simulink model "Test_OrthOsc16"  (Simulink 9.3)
settings: Solver=VariableStepAuto  StartTime=0.0  StopTime=0.4  RelTol=1e-3
InitFcn:
  | Test_LibVishia_Ctrl.TestOrthOsc_init()
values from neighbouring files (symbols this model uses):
  Orth_fb = 0    [stimuli_OrthBandpass.m]
  Orth_fqA = 50    [stimuli_OrthBandpass.m]
  Orth_fqB = 0    [stimuli_OrthBandpass.m]
  Orth_k0AB = 1    [stimuli_OrthBandpass.m]
  Orth_kA = 0.1    [stimuli_OrthBandpass.m]
  Orth_kB = 0    [stimuli_OrthBandpass.m]
  Tfq = 0.020    (= 0.02)    [TestOrthOsc_init.m]
  Tstep = 0.000050    (= 5e-05)    [TestOrthOsc_init.m]    (also in Test_PIDctrl_init.m = 0.0001)
libraries: libVishia_CtrlSfn x23, libVishia_Conv x16, libVishia_Ctrl x10, libVishia_Inspc x5, simulink x2

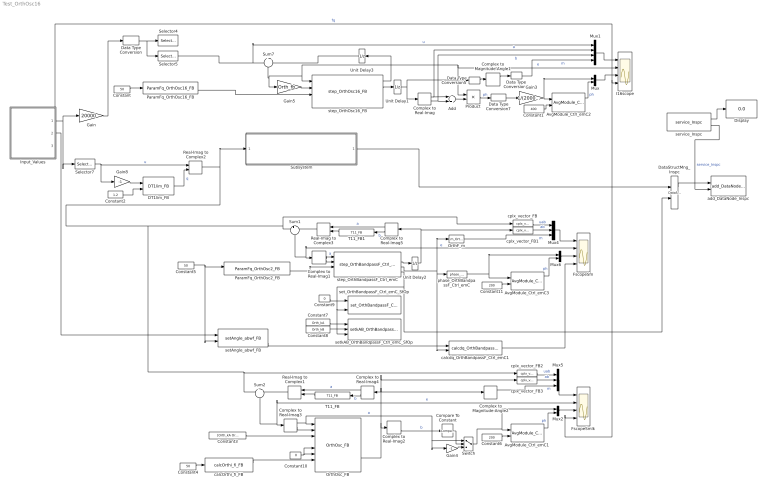
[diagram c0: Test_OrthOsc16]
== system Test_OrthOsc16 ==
  Add : Sum
  AvgModule_Ctrl_emC1 : libVishia_CtrlSfn/AvgModule_Ctrl_emC  SystemSampleTime=-1
  AvgModule_Ctrl_emC2 : libVishia_CtrlSfn/AvgModule_Ctrl_emC  SystemSampleTime=-1
  AvgModule_Ctrl_emC3 : libVishia_CtrlSfn/AvgModule_Ctrl_emC  SystemSampleTime=-1
  Compare To Constant : simulink/Logic and Bit Operations/Compare To Constant  relop=>=  const=0  OutDataTypeStr=boolean
  Complex to Magnitude-Angle1 : ComplexToMagnitudeAngle
  Complex to Magnitude-Angle2 : ComplexToMagnitudeAngle
  Complex to Real-Imag{,1..5} (6 alike) : ComplexToRealImag
  Constant : Constant  Value=50  OutDataTypeStr=single
  Constant1 : Constant  Value=400  OutDataTypeStr=single
  Constant10 : Constant  Value=0  OutDataTypeStr=boolean
  Constant11 : Constant  Value=200  OutDataTypeStr=single
  Constant2 : Constant  Value=1.2  OutDataTypeStr=single
  Constant3 : Constant  Value=[Orth_kA Orth_kB]  OutDataTypeStr=single
  Constant4 : Constant  Value=50  OutDataTypeStr=single
  Constant5 : Constant  Value=50  OutDataTypeStr=single
  Constant6 : Constant  Value=200  OutDataTypeStr=single
  Constant7 : Constant  Value=Orth_kA  OutDataTypeStr=single
  Constant8 : Constant  Value=Orth_kB  OutDataTypeStr=single
  Constant9 : Constant  Value=0  OutDataTypeStr=boolean
  DT1lim_FB : libVishia_Ctrl/DT1lim_FB  T1=0.0002  Td=0.02 / (2*pi)  Tstep=Tstep
  Data Type Conversion : DataTypeConversion  OutDataTypeStr=int16
  Data Type Conversion5 : DataTypeConversion  OutDataTypeStr=single
  Data Type Conversion6 : DataTypeConversion  OutDataTypeStr=int16
  Data Type Conversion7 : DataTypeConversion  OutDataTypeStr=single
  DataStructMng_Inspc : libVishia_Inspc/DataStructMng_Inspc  dirGenSource=''  typeData='Test_OrthBandpass'  inherit=off  chain=off  inputs=|
      | =f32: F32_Test_OrthBandpass;
      | =f: OrthBandpassF_Ctrl_emC;
  Display : Display
  FscopeSfn : Scope  NumInputPorts=4
  FscopeSmlk : Scope  NumInputPorts=4
  Gain : Gain  Gain=20000
  Gain3 : Gain  Gain=1/(20000*20000)
  Gain4 : Gain  Gain=-1
  Gain5 : Gain  Gain=Orth_fb
  Gain8 : Gain  Gain=-1
  I16scope : Scope  NumInputPorts=4
  Input_Values : Subsystem
  Mux : Mux  Inputs=2
  Mux1 : Mux
  Mux2 : Mux  Inputs=2
  Mux4 : Mux  Inputs=3
  Mux5 : Mux  Inputs=3
  Mux6 : Mux  Inputs=2
  OrthF_m : libVishia_CtrlSfn/m_OrthBandpass_Ctrl_emC  SystemSampleTime=-1
  OrthOsc_FB : libVishia_Ctrl/OrthOsc_FB
  ParamFq_OrthOsc16_FB : libVishia_CtrlSfn/ParamFq_OrthOsc16_FB  identObj=123  Tstep=16*Tstep  TstepOrth=Tstep  m_nom=100
  ParamFq_OrthOsc2_FB : libVishia_CtrlSfn/ParamFq_OrthOsc2_FB  identObj=123  Tstep=16*Tstep  TstepOrth=Tstep  m_nom=1.0
  Product : Product
  Real-Imag to Complex1 : RealImagToComplex
  Real-Imag to Complex2 : RealImagToComplex
  Real-Imag to Complex3 : RealImagToComplex
  Selector4 : Selector  IndexMode=Zero-based  InputPortWidth=2  IndexOptions=Index vector (dialog)  Indices=[0]  OutputSizes=1
  Selector5 : Selector  IndexMode=Zero-based  InputPortWidth=2  IndexOptions=Index vector (dialog)  Indices=[1]  OutputSizes=1
  Selector7 : Selector  IndexMode=Zero-based  InputPortWidth=2  IndexOptions=Index vector (dialog)  Indices=[1]  OutputSizes=1
  Subsystem : Subsystem
  Sum1 : Sum  Inputs=+|-
  Sum2 : Sum  Inputs=+|-
  Sum7 : Sum  Inputs=+|-
  Switch : Switch  Criteria=u2 > Threshold
  T11_FB : libVishia_Ctrl/T11_FB  T1=0.0002  y0=0  Tstep=Tstep
  T11_FB1 : libVishia_Ctrl/T11_FB  T1=0.0002  y0=0  Tstep=Tstep
  Unit Delay1 : UnitDelay  SampleTime=-1  HasFrameUpgradeWarning=on
  Unit Delay2 : UnitDelay  SampleTime=-1  HasFrameUpgradeWarning=on
  Unit Delay3 : UnitDelay  SampleTime=-1  HasFrameUpgradeWarning=on
  add_DataNode_Inspc : libVishia_Inspc/add_DataNode_Inspc  name1Refl='main'  name2Refl='_data'
  calcOrthi_fi_FB : libVishia_Ctrl/calcOrthi_fi_FB  Tstep=Tstep
  calcdq_OrthBandpassF_Ctrl_emC1 : libVishia_CtrlSfn/calcdq_OrthBandpassF_Ctrl_emC1  SystemSampleTime=-1
  cplx_vector_FB{,1..3} (4 alike) : libVishia_Conv/cplx_vector_FB  SystemSampleTime=-1
  phase_OrthBandpassF_Ctrl_emC : libVishia_CtrlSfn/phase_OrthBandpassF_Ctrl_emC  SystemSampleTime=-1
  service_Inspc : libVishia_Inspc/service_Inspc  Tstep=Tstep  IpPort='UDP:0.0.0.0:60094'
  setAngle_abwf_FB : libVishia_CtrlSfn/setAngle_abwf_FB  identObj=123  Tstep=Tstep
  set_OrthBandpassF_Ctrl_emC_SfOp : libVishia_CtrlSfn/set_OrthBandpassF_Ctrl_emC_SfOp  SystemSampleTime=-1
  setkAB_OrthBandpassF_Ctrl_emC_SfOp : libVishia_CtrlSfn/setkAB_OrthBandpassF_Ctrl_emC_SfOp  SystemSampleTime=-1
  step_OrthBandpassF_Ctrl_emC : libVishia_CtrlSfn/step_OrthBandpassF_Ctrl_emC  kA=1.0  kB=0
  step_OrthOsc16_FB : libVishia_CtrlSfn/step_OrthOsc16_FB  kA=Orth_kA  kB=Orth_kB
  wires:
  ParamFq_OrthOsc16_FB/2 -> step_OrthOsc16_FB/3
  Input_Values/1(Out1) -> Selector7/1, Gain/1
  Data Type Conversion/1 -> Selector5/1, Selector4/1
  Selector5/1 -> Sum7/1, Mux1/1  "u"
  Constant/1 -> ParamFq_OrthOsc16_FB/1
  Input_Values/2(Out2) -> setAngle_abwf_FB/1
  step_OrthOsc16_FB/2 -> Unit Delay1/1
  Add/1 -> Product/2
  Sum7/1 -> Gain5/1, step_OrthOsc16_FB/1, I16scope/2, Product/1  "e"
  Gain/1 -> Data Type Conversion/1
  Input_Values/3(Out3) -> FscopeSmlk/4, I16scope/4  "fq"
  Constant3/1 -> OrthOsc_FB/3
  calcOrthi_fi_FB/1 -> OrthOsc_FB/7
  Constant4/1 -> calcOrthi_fi_FB/1
  OrthOsc_FB/3 -> Complex to Magnitude-Angle2/1, cplx_vector_FB3/1, Complex to Real-Imag4/1, Complex to Real-Imag2/1
  Mux5/1 -> FscopeSmlk/1
  Complex to Real-Imag2/2 -> Compare To Constant/1  "b"
  Selector7/1 -> Real-Imag to Complex2/1, Gain8/1  "u"
  Switch/1 -> Mux2/1, AvgModule_Ctrl_emC1/1
  Sum2/1 -> FscopeSmlk/2, Complex to Real-Imag3/1  "e"
  Constant6/1 -> AvgModule_Ctrl_emC1/2
  AvgModule_Ctrl_emC1/1 -> Mux2/2  "ph"
  Product/1 -> Data Type Conversion7/1  "ph"
  Complex to Real-Imag/2 -> Mux1/3, Add/2  "b"
  Complex to Real-Imag/1 -> Mux1/2, Add/1  "a"
  Mux1/1 -> I16scope/1
  Unit Delay1/1 -> Data Type Conversion5/1, Complex to Real-Imag/1
  Data Type Conversion5/1 -> Complex to Magnitude-Angle1/1
  Complex to Magnitude-Angle1/1 -> Data Type Conversion6/1
  Data Type Conversion6/1 -> Mux1/4  "m"
  Complex to Magnitude-Angle2/1 -> Mux5/3  "m"
  Data Type Conversion7/1 -> Gain3/1
  Constant1/1 -> AvgModule_Ctrl_emC2/2
  Gain3/1 -> Mux/1, AvgModule_Ctrl_emC2/1
  AvgModule_Ctrl_emC2/1 -> Mux/2  "ph"
  Mux/1 -> I16scope/3
  Mux2/1 -> FscopeSmlk/3
  Compare To Constant/1 -> Switch/2
  Gain4/1 -> Switch/3
  Gain5/1 -> step_OrthOsc16_FB/2
  Complex to Real-Imag3/2 -> OrthOsc_FB/2
  DT1lim_FB/2 -> Real-Imag to Complex2/2  "q"
  Gain8/1 -> DT1lim_FB/1
  Real-Imag to Complex2/1 -> Subsystem/1(In1), Sum1/1, cplx_vector_FB/1, cplx_vector_FB2/1, Sum2/1
  Complex to Real-Imag3/1 -> Gain4/1, Switch/1, OrthOsc_FB/1  "a"
  Complex to Real-Imag4/2 -> T11_FB/1  "b"
  T11_FB/1 -> Real-Imag to Complex1/2
  Complex to Real-Imag4/1 -> Real-Imag to Complex1/1  "a"
  Real-Imag to Complex1/1 -> Sum2/2
  Subsystem/1(Out1) -> DataStructMng_Inspc/1
  DataStructMng_Inspc/1 -> add_DataNode_Inspc/1
  service_Inspc/1 -> Display/1
  service_Inspc/2 -> add_DataNode_Inspc/2  "service_Inspc"
  Constant2/1 -> DT1lim_FB/2
  ParamFq_OrthOsc2_FB/2 -> step_OrthBandpassF_Ctrl_emC/3
  Constant5/1 -> setAngle_abwf_FB/2, ParamFq_OrthOsc2_FB/1
  Complex to Real-Imag1/1 -> step_OrthBandpassF_Ctrl_emC/1  "a"
  Complex to Real-Imag1/2 -> step_OrthBandpassF_Ctrl_emC/2
  Sum1/1 -> FscopeSfn/2, Complex to Real-Imag1/1  "e"
  step_OrthBandpassF_Ctrl_emC/2 -> Unit Delay2/1
  Unit Delay2/1 -> cplx_vector_FB1/1, Complex to Real-Imag5/1
  Mux4/1 -> FscopeSfn/1
  setAngle_abwf_FB/3 -> calcdq_OrthBandpassF_Ctrl_emC1/1
  cplx_vector_FB/1 -> Mux4/1  "uab"
  cplx_vector_FB1/1 -> Mux4/2  "ab"
  step_OrthBandpassF_Ctrl_emC/4 -> setkAB_OrthBandpassF_Ctrl_emC_SfOp/3, set_OrthBandpassF_Ctrl_emC_SfOp/3, DataStructMng_Inspc/2
  OrthF_m/1 -> Mux4/3  "m"
  step_OrthBandpassF_Ctrl_emC/3 -> phase_OrthBandpassF_Ctrl_emC/1, calcdq_OrthBandpassF_Ctrl_emC1/2, OrthF_m/1
  calcdq_OrthBandpassF_Ctrl_emC1/1 -> FscopeSfn/4
  cplx_vector_FB2/1 -> Mux5/1  "uab"
  cplx_vector_FB3/1 -> Mux5/2  "ab"
  Complex to Real-Imag5/1 -> Real-Imag to Complex3/1  "a"
  Complex to Real-Imag5/2 -> T11_FB1/1  "b"
  T11_FB1/1 -> Real-Imag to Complex3/2
  Real-Imag to Complex3/1 -> Sum1/2
  Constant7/1 -> setkAB_OrthBandpassF_Ctrl_emC_SfOp/1
  Constant8/1 -> setkAB_OrthBandpassF_Ctrl_emC_SfOp/2
  Constant9/1 -> set_OrthBandpassF_Ctrl_emC_SfOp/1
  Constant10/1 -> OrthOsc_FB/5, OrthOsc_FB/6
  phase_OrthBandpassF_Ctrl_emC/1 -> Mux6/1, AvgModule_Ctrl_emC3/1
  Mux6/1 -> FscopeSfn/3
  AvgModule_Ctrl_emC3/1 -> Mux6/2  "ph"
  Constant11/1 -> AvgModule_Ctrl_emC3/2
  step_OrthOsc16_FB/1 -> Unit Delay3/1
  Unit Delay3/1 -> Sum7/2

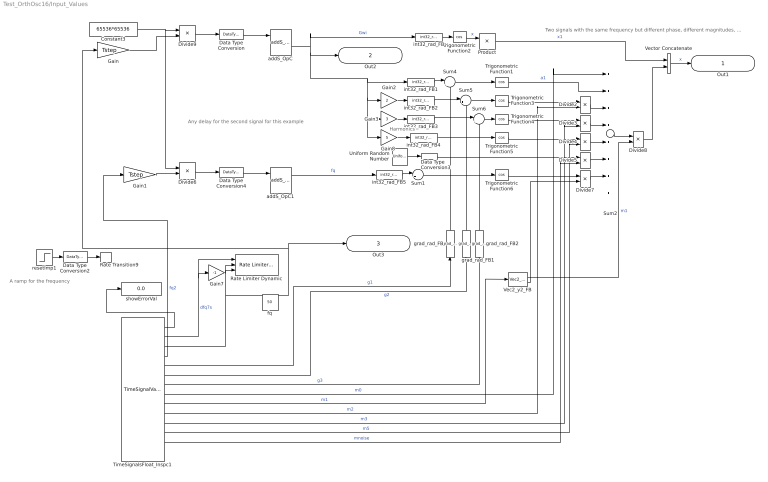
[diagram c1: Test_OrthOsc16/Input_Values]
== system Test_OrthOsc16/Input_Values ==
  note: A ramp for the frequency
  note: Two signals with the same frequency but different phase, different magnitudes, one signal has harmonics.
  note: Harmonics
  note: Any delay for the second signal for this example
  Constant3 : Constant  Value=65536*65536  OutDataTypeStr=single
  Data Type Conversion : DataTypeConversion  OutDataTypeStr=int32
  Data Type Conversion2 : DataTypeConversion  OutDataTypeStr=single
  Data Type Conversion3 : DataTypeConversion  OutDataTypeStr=single
  Data Type Conversion4 : DataTypeConversion  OutDataTypeStr=int32
  Divide{2..9} (8 alike) : Product  Inputs=**
  Gain : Gain  Gain=Tstep
  Gain1 : Gain  Gain=Tstep
  Gain2 : Gain  Gain=2
  Gain3 : Gain  Gain=3
  Gain7 : Gain  Gain=-1
  Gain8 : Gain  Gain=5
  Product : Product
  Rate Limiter Dynamic : simulink/Discontinuities/Rate Limiter Dynamic
  Rate Transition9 : RateTransition  Integrity=off  Deterministic=off  OutPortSampleTime=Tfq
  Sum{1,4..6} (4 alike) : Sum  Inputs=|++
  Sum2 : Sum  Inputs=++++++++
  TimeSignalsFloat_Inspc1 : libVishia_Inspc/TimeSignalValue_Inspc  Description=|  Tstep=Tstep  filepath=timeSignalFilepath  nameRefl='stimuli'  nrofStimuli=25  varDef=|
      | A combined stimuli and inspector function block.
      | Stimuli file path: file contains stimuli in form:
      |   %time:0: stimuli.namex = 5000.0, stimuli.namey = 50.0 -10; 
      | Name in reflection-tree: Name of this function block for stimuli and inspector access
      | name1..12: output type and name, base type is single always.
      | C2:namexy  A complex array of 2 elements
      | 6:namexy An array of 6 elements (max).
      | C:namexy  A 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
      | dfq7s:F;
      | fq:F;
      | fq2:F;
      | g1:F;
      | g2:F;
      | g3:F;
      | m0:F;
      | m1:F*2;
      | m2:F;
      | m3:F;
      | m5:F;
      | mnoise: F;
  Trigonometric Function{1..6} (6 alike) : Trigonometry  Operator=cos
  Uniform Random Number : UniformRandomNumber  SampleTime=Tstep
  Vec2_y2_FB : libVishia_Conv/Vec2_y2_FB  SystemSampleTime=-1
  Vector Concatenate : Concatenate
  addS_OpC : libVishia_Ctrl/addS_OpC  init=0  Tstep=-1
  addS_OpC1 : libVishia_Ctrl/addS_OpC  init=0  Tstep=-1
  fq : Constant  Value=50  OutDataTypeStr=single
  grad_rad_FB : libVishia_Conv/grad_rad_FB  SystemSampleTime=-1
  grad_rad_FB1 : libVishia_Conv/grad_rad_FB  SystemSampleTime=-1
  grad_rad_FB2 : libVishia_Conv/grad_rad_FB  SystemSampleTime=-1
  int32_rad_FB{,1..5} (6 alike) : libVishia_Conv/int32_rad_FB  SystemSampleTime=-1
  resetImp1 : Step  Time=0.1  Before=0.995  After=1.2  SampleTime=Tfq
  showErrorVal : Display
  Out1 : Outport  OutDataTypeStr=single  PortDimensions=2
  Out2 : Outport  Port=2  OutDataTypeStr=int32  PortDimensions=1
  Out3 : Outport  Port=3  OutDataTypeStr=single  PortDimensions=1
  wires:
  TimeSignalsFloat_Inspc1/4 -> Gain1/1  "fq2"
  Constant3/1 -> Divide6/1, Divide9/1
  int32_rad_FB/1 -> Trigonometric Function2/1
  Trigonometric Function2/1 -> Product/1  "x"
  Divide9/1 -> Data Type Conversion/1
  int32_rad_FB1/1 -> Sum4/1
  Product/1 -> Vector Concatenate/1  "x1"
  Trigonometric Function1/1 -> Sum2/2  "a1"
  Gain/1 -> Divide9/2
  Data Type Conversion/1 -> addS_OpC/1
  Data Type Conversion2/1 -> Rate Transition9/1
  Gain3/1 -> int32_rad_FB3/1
  Gain2/1 -> int32_rad_FB2/1
  int32_rad_FB2/1 -> Sum5/1
  int32_rad_FB3/1 -> Sum6/1
  Trigonometric Function3/1 -> Divide2/1
  Divide2/1 -> Sum2/3
  Trigonometric Function4/1 -> Divide3/1
  Divide3/1 -> Sum2/4
  Divide8/1 -> Vector Concatenate/2
  Rate Transition9/1 -> ?
  resetImp1/1 -> Data Type Conversion2/1
  Vector Concatenate/1 -> Out1/1  "x"
  addS_OpC/2 -> int32_rad_FB/1, int32_rad_FB1/1, Gain8/1, Gain3/1, Gain2/1, Out2/1  "Gwi"
  Vec2_y2_FB/1 -> Divide8/2  "m1"
  TimeSignalsFloat_Inspc1/10 -> Divide2/2  "m2"
  TimeSignalsFloat_Inspc1/11 -> Divide3/2  "m3"
  Sum6/1 -> Trigonometric Function4/1
  TimeSignalsFloat_Inspc1/5 -> grad_rad_FB/1  "g1"
  TimeSignalsFloat_Inspc1/6 -> grad_rad_FB1/1  "g2"
  TimeSignalsFloat_Inspc1/7 -> grad_rad_FB2/1  "g3"
  Sum5/1 -> Trigonometric Function3/1
  Sum4/1 -> Trigonometric Function1/1
  grad_rad_FB/1 -> Sum4/2
  grad_rad_FB1/1 -> Sum5/2
  grad_rad_FB2/1 -> Sum6/2
  TimeSignalsFloat_Inspc1/3 -> Out3/1, Gain/1, Rate Limiter Dynamic/2
  TimeSignalsFloat_Inspc1/2 -> Gain7/1, Rate Limiter Dynamic/1  "dfq7s"
  Gain7/1 -> Rate Limiter Dynamic/3
  Gain8/1 -> int32_rad_FB4/1
  Trigonometric Function5/1 -> Divide4/1
  Divide4/1 -> Sum2/5
  int32_rad_FB4/1 -> Trigonometric Function5/1
  TimeSignalsFloat_Inspc1/12 -> Divide4/2  "m5"
  TimeSignalsFloat_Inspc1/8 -> Sum2/1  "m0"
  TimeSignalsFloat_Inspc1/1 -> showErrorVal/1
  TimeSignalsFloat_Inspc1/9 -> Vec2_y2_FB/1  "m1"
  Divide5/1 -> Sum2/6
  Uniform Random Number/1 -> Data Type Conversion3/1
  TimeSignalsFloat_Inspc1/13 -> Divide5/2  "mnoise"
  Data Type Conversion3/1 -> Divide5/1
  Gain1/1 -> Divide6/2
  Divide6/1 -> Data Type Conversion4/1
  Data Type Conversion4/1 -> addS_OpC1/1
  Sum1/1 -> Trigonometric Function6/1
  int32_rad_FB5/1 -> Sum1/1
  addS_OpC1/1 -> int32_rad_FB5/1  "fq"
  Trigonometric Function6/1 -> Divide7/1
  Divide7/1 -> Sum2/7
  Vec2_y2_FB/2 -> Divide7/2
  Sum2/1 -> Divide8/1

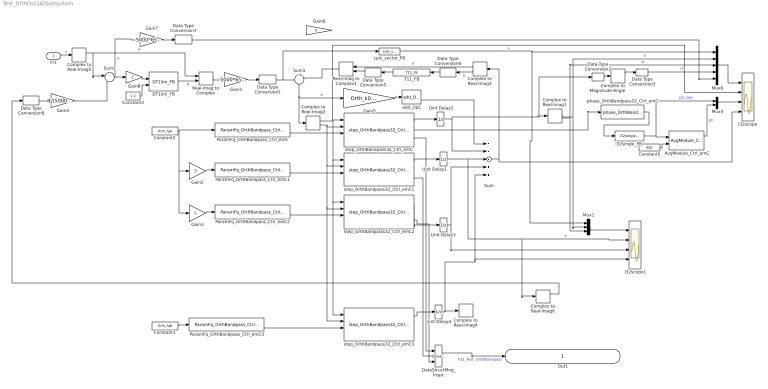
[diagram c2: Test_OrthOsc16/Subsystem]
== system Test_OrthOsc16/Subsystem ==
  In1 : Inport  OutDataTypeStr=single
  AvgModule_Ctrl_emC : libVishia_CtrlSfn/AvgModule_Ctrl_emC  SystemSampleTime=-1
  Complex to Magnitude-Angle : ComplexToMagnitudeAngle
  Complex to Real-Imag{1..6} (6 alike) : ComplexToRealImag
  Constant1 : Constant  Value=Orth_fqB  OutDataTypeStr=single
  Constant2 : Constant  Value=Orth_fqA  OutDataTypeStr=single
  Constant3 : Constant  Value=1.2  OutDataTypeStr=int32
  Constant5 : Constant  Value=400  OutDataTypeStr=single
  DT1lim_FB : libVishia_Ctrl/DT1lim_FB  T1=0.001  Td=0.02 / (2*pi)  Tstep=Tstep
  Data Type Conversion{1,3,5,7} (4 alike) : DataTypeConversion  OutDataTypeStr=int32
  Data Type Conversion2 : DataTypeConversion  OutDataTypeStr=single
  Data Type Conversion6 : DataTypeConversion  OutDataTypeStr=single
  Data Type Conversion8 : DataTypeConversion  OutDataTypeStr=single
  DataStructMng_Inspc : libVishia_Inspc/DataStructMng_Inspc  dirGenSource=''  typeData='F32_Test_OrthBandpass'  inherit=off  chain=off  inputs=|
      | =f1: OrthBandpass32_Ctrl_emC;
      | =f3: OrthBandpass32_Ctrl_emC;
      | =f5: OrthBandpass32_Ctrl_emC;
  Gain1 : Gain  Gain=5000*65536
  Gain2 : Gain  Gain=3
  Gain3 : Gain  Gain=5
  Gain4 : Gain  Gain=1/(5000*65536)
  Gain5 : Gain  Gain=Orth_k0AB*Tstep
  Gain6 : Gain  Gain=0
  Gain7 : Gain  Gain=5000*65536
  Gain8 : Gain  Gain=-1
  I32scope : Scope  NumInputPorts=4
  I32scope1 : Scope  NumInputPorts=4
  Mux1 : Mux  Inputs=3
  Mux4 : Mux  Inputs=2
  Mux8 : Mux  Inputs=5
  ParamFq_OrthBandpass_Ctrl_emC{,1..3} (4 alike) : libVishia_CtrlSfn/ParamFq_OrthBandpass_Ctrl_emC  identObj=123  Tstep=16*Tstep  TstepOrth=Tstep  m_nom=100
  Real-Imag to Complex : RealImagToComplex
  Real-Imag to Complex1 : RealImagToComplex
  Sum : Sum  Inputs=+++++
  Sum1 : Sum  Inputs=+|-
  Sum2 : Sum  Inputs=|+-
  T11_FB : libVishia_Ctrl/T11_FB  T1=0.001  y0=0  Tstep=Tstep
  Unit Delay{1..4} (4 alike) : UnitDelay  SampleTime=-1  HasFrameUpgradeWarning=on
  add_OpC : libVishia_Ctrl/add_OpC  y0=0  Tstep=-1
  cplx_vector_FB : libVishia_Conv/cplx_vector_FB  SystemSampleTime=-1
  i32single_FB : libVishia_Conv/i32single_FB  ynom=1.0
  phase_OrthBandpass32_Ctrl_emC : libVishia_CtrlSfn/phase_OrthBandpass32_Ctrl_emC  SystemSampleTime=-1
  step_OrthBandpass32_Ctrl_emC : libVishia_CtrlSfn/step_OrthBandpass32_Ctrl_emC  ident=0  kA=Orth_kA  kB=Orth_kB
  step_OrthBandpass32_Ctrl_emC1 : libVishia_CtrlSfn/step_OrthBandpass32_Ctrl_emC  ident=0  kA=Orth_kA3  kB=Orth_kB3
  step_OrthBandpass32_Ctrl_emC2 : libVishia_CtrlSfn/step_OrthBandpass32_Ctrl_emC  ident=0  kA=Orth_kA3  kB=Orth_kB3
  step_OrthBandpass32_Ctrl_emC3 : libVishia_CtrlSfn/step_OrthBandpass32_Ctrl_emC  ident=0  kA=Orth_kA  kB=Orth_kB
  Out1 : Outport  OutDataTypeStr=uint32  PortDimensions=1
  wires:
  Unit Delay2/1 -> Sum/2, Data Type Conversion2/1, Complex to Real-Imag1/1
  Complex to Magnitude-Angle/1 -> Data Type Conversion3/1
  step_OrthBandpass32_Ctrl_emC/2 -> phase_OrthBandpass32_Ctrl_emC/1
  Mux8/1 -> I32scope/1
  Complex to Real-Imag1/1 -> Mux1/2, Mux8/2  "a"
  Constant2/1 -> Gain3/1, Gain2/1, ParamFq_OrthBandpass_Ctrl_emC/1
  Data Type Conversion2/1 -> Complex to Magnitude-Angle/1
  Complex to Real-Imag1/2 -> Mux1/3, Mux8/3  "b"
  Constant5/1 -> AvgModule_Ctrl_emC/2
  i32single_FB/1 -> Mux4/1, AvgModule_Ctrl_emC/1  "ph_raw"
  AvgModule_Ctrl_emC/1 -> Mux4/2  "ph"
  ParamFq_OrthBandpass_Ctrl_emC/2 -> step_OrthBandpass32_Ctrl_emC/3
  Data Type Conversion1/1 -> cplx_vector_FB/1, Sum1/1
  Data Type Conversion3/1 -> Mux8/4  "m"
  step_OrthBandpass32_Ctrl_emC/1 -> Unit Delay2/1
  phase_OrthBandpass32_Ctrl_emC/1 -> i32single_FB/1
  Mux4/1 -> I32scope/3
  ? -> ?  "fq"
  In1/1 -> Complex to Real-Imag5/1  "u"
  ParamFq_OrthBandpass_Ctrl_emC1/2 -> step_OrthBandpass32_Ctrl_emC1/3
  Gain2/1 -> ParamFq_OrthBandpass_Ctrl_emC1/1
  Sum/1 -> I32scope/4, Complex to Real-Imag3/1
  step_OrthBandpass32_Ctrl_emC1/1 -> Unit Delay1/1
  Unit Delay1/1 -> Complex to Real-Imag6/1, I32scope1/2, Sum/3  "a"
  Unit Delay3/1 -> Sum/4, I32scope1/3
  Gain3/1 -> ParamFq_OrthBandpass_Ctrl_emC2/1
  ParamFq_OrthBandpass_Ctrl_emC2/2 -> step_OrthBandpass32_Ctrl_emC2/3
  step_OrthBandpass32_Ctrl_emC2/1 -> Unit Delay3/1
  step_OrthBandpass32_Ctrl_emC/3 -> DataStructMng_Inspc/1
  step_OrthBandpass32_Ctrl_emC1/3 -> DataStructMng_Inspc/2
  step_OrthBandpass32_Ctrl_emC2/3 -> DataStructMng_Inspc/3
  DataStructMng_Inspc/1 -> Out1/1  "F32_Test_OrthBandpass"
  Complex to Real-Imag2/2 -> step_OrthBandpass32_Ctrl_emC3/2, step_OrthBandpass32_Ctrl_emC2/2, step_OrthBandpass32_Ctrl_emC1/2, step_OrthBandpass32_Ctrl_emC/2
  Complex to Real-Imag2/1 -> step_OrthBandpass32_Ctrl_emC3/1, step_OrthBandpass32_Ctrl_emC2/1, step_OrthBandpass32_Ctrl_emC1/1, step_OrthBandpass32_Ctrl_emC/1, I32scope/2  "e"
  ParamFq_OrthBandpass_Ctrl_emC3/2 -> step_OrthBandpass32_Ctrl_emC3/3
  Constant1/1 -> ParamFq_OrthBandpass_Ctrl_emC3/1
  step_OrthBandpass32_Ctrl_emC3/1 -> Unit Delay4/1
  Unit Delay4/1 -> Sum/5, I32scope1/4, Complex to Real-Imag4/1
  Mux1/1 -> I32scope1/1
  Sum1/1 -> Complex to Real-Imag2/1, Gain5/1  "e"
  cplx_vector_FB/1 -> Mux1/1, Mux8/1
  Constant3/1 -> DT1lim_FB/2
  Gain8/1 -> DT1lim_FB/1
  Complex to Real-Imag5/1 -> Real-Imag to Complex/1, Sum2/1  "a"
  DT1lim_FB/2 -> Real-Imag to Complex/2  "q"
  Gain1/1 -> Data Type Conversion1/1
  Real-Imag to Complex/1 -> Gain1/1
  Sum2/1 -> Gain7/1, Gain8/1  "e"
  Gain4/1 -> Sum2/2
  Complex to Real-Imag6/1 -> Data Type Conversion8/1
  add_OpC/2 -> Sum/1
  Gain5/1 -> add_OpC/1
  Complex to Real-Imag3/1 -> Real-Imag to Complex1/1  "a"
  T11_FB/1 -> Data Type Conversion5/1
  Complex to Real-Imag3/2 -> Data Type Conversion6/1  "b"
  Real-Imag to Complex1/1 -> Sum1/2
  Data Type Conversion6/1 -> T11_FB/1
  Data Type Conversion5/1 -> Real-Imag to Complex1/2
  Gain7/1 -> Data Type Conversion7/1
  Data Type Conversion7/1 -> Mux8/5
  Data Type Conversion8/1 -> Gain4/1
